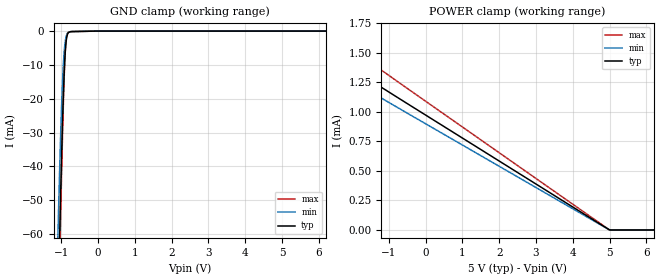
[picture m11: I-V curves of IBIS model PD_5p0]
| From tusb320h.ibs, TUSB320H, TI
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|   Model
[Model]   PD_5p0
Model_type   Input
Vinl = 1.5
Vinh = 3.5
|   typ   min   max
C_comp   0.475pF   0.451pF   0.489pF
[Voltage Range]   5   4.999   5.001
[Temperature Range]   27   105   -40
[Power Clamp Reference]   5   4.999   5.001
[GND Clamp Reference]   0   0   0
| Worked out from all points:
|   GND clamp passes 1 mA (typ) near -0.83 V on its own axis
|   POWER clamp passes 1 mA (typ) near -0.13 V on its own axis
[GND Clamp]
|   Voltage   I(typ)   I(min)   I(max)
-5V       -2.345A    -2.242A    -2.422A
-1.085V   -81.56mA   -58.86mA   -91.13mA
-1.04V    -59.74mA   -40.17mA   -67.54mA
-1.025V   -52.78mA   -34.45mA   -59.92mA
-995mV    -39.5mA    -24.01mA   -45.2mA
-965mV    -27.39mA   -15.29mA   -31.47mA
-935mV    -17.01mA   -8.722mA   -19.3mA
-905mV    -9.061mA   -4.446mA   -9.673mA
-890mV    -6.182mA   -3.071mA   -6.182mA
-860mV    -2.558mA   -1.422mA   -2.076mA
-800mV    -426.7uA   -357.2uA   -285.7uA
10V       0A         0A         0A
[POWER Clamp]
|   Voltage   I(typ)   I(min)   I(max)
-5V       1.957mA    1.593A     2.195mA
-3.77V    1.715mA    896.5mA    1.923mA
-3.335V   1.63mA     652.3mA    1.827mA
-2.69V    1.503mA    296.2mA    1.684mA
-2V       1.367mA    2.466mA    1.532mA
-1.91V    1.349mA    1.328mA    1.512mA
-1.25V    1.219mA    1.127mA    1.366mA
4.99V     1.934uA    1.604uA    2.388uA
10V       0A         0A         0A
